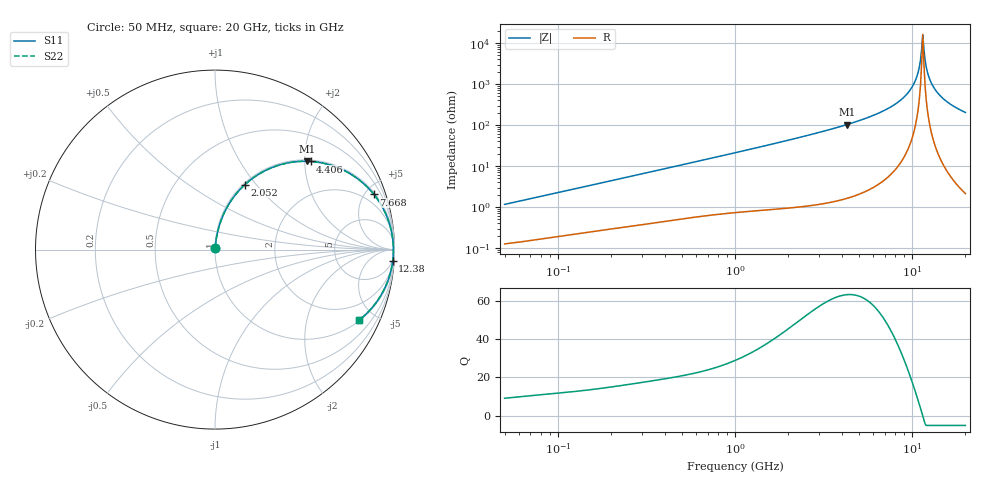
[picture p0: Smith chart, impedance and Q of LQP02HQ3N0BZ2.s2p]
!Murata Part Number: LQP02HQ3N0BZ2
!These Parameters are Measured in Series Mode Connection
!  o--[Z]--o
!Port1  Port2
!  o-------o
!Freq. Start=50[MHz] Stop=20[GHz], 401[Steps]
# Hz S RI R 50
!Freq.(Hz) S11(Real) S11(Imag) S21(Real) S21(Imag) S12(Real) S12(Imag) S22(Real) S22(Imag)
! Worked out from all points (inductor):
!   401 points, 50 MHz to 20 GHz, reference 50 ohm
!   read as one part in series: L = 3.65 nH near 51.52 MHz
!   highest Q = 63.1 at 4.276 GHz (marker M1), where L = 3.82 nH
!   self-resonance near 11.49 GHz
!   S11 on the Smith chart (normalised r, x): 50 MHz: 1.00, +0.02; 2.052 GHz: 1.02, +0.88; 4.406 GHz: 1.03, +2.14; 7.668 GHz: 1.13, +5.71; 12.38 GHz: 4, -31; 20 GHz: 1.04, -4.08
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5e7  0.00139 0.0115  0.9986 -0.0115  0.9986 -0.0115  0.00139 0.0115
1.364002e8  0.00323 0.0302  0.9968 -0.0302  0.9968 -0.0302  0.00323 0.0302
3.721004e8  0.0105 0.0789  0.9895 -0.0789  0.9895 -0.0789  0.0105 0.0789
1e9  0.049 0.1992  0.951 -0.1992  0.951 -0.1992  0.049 0.1992
2.05233e9  0.1675 0.3627  0.8325 -0.3627  0.8325 -0.3627  0.1675 0.3627
2.728004e9  0.2677 0.4337  0.7323 -0.4337  0.7323 -0.4337  0.2677 0.4337
4.275624e9  0.5129 0.492  0.4871 -0.492  0.4871 -0.492  0.5129 0.492
4.405649e9  0.5325 0.4911  0.4675 -0.4911  0.4675 -0.4911  0.5325 0.4911
7.442007e9  0.8699 0.3256  0.1301 -0.3256  0.1301 -0.3256  0.8699 0.3256
7.668323e9  0.8853 0.3074  0.1147 -0.3074  0.1147 -0.3074  0.8853 0.3074
9.041845e9  0.9539 0.1931  0.0461 -0.1931  0.0461 -0.1931  0.9539 0.1931
1.004137e10  0.9808 0.1111  0.0192 -0.1111  0.0192 -0.1111  0.9808 0.1111
1.066139e10  0.9897 0.0622  0.0103 -0.0622  0.0103 -0.0622  0.9897 0.0622
1.098561e10  0.9923 0.0375  0.00766 -0.0375  0.00766 -0.0375  0.9923 0.0375
1.115139e10  0.9932 0.0251  0.00683 -0.0251  0.00683 -0.0251  0.9932 0.0251
1.149051e10  0.9939 0.000173  0.00611 -0.000173  0.00611 -0.000173  0.9939 0.000173
1.183995e10  0.9934 -0.0247  0.00664 0.0247  0.00664 0.0247  0.9934 -0.0247
1.201863e10  0.9926 -0.0372  0.00737 0.0372  0.00737 0.0372  0.9926 -0.0372
1.238412e10  0.9902 -0.062  0.00978 0.062  0.00978 0.062  0.9902 -0.062
1.314879e10  0.9817 -0.1109  0.0183 0.1109  0.0183 0.1109  0.9817 -0.1109
1.460232e10  0.9553 -0.1934  0.0447 0.1934  0.0447 0.1934  0.9553 -0.1934
2e10  0.8034 -0.3922  0.1966 0.3922  0.1966 0.3922  0.8034 -0.3922
